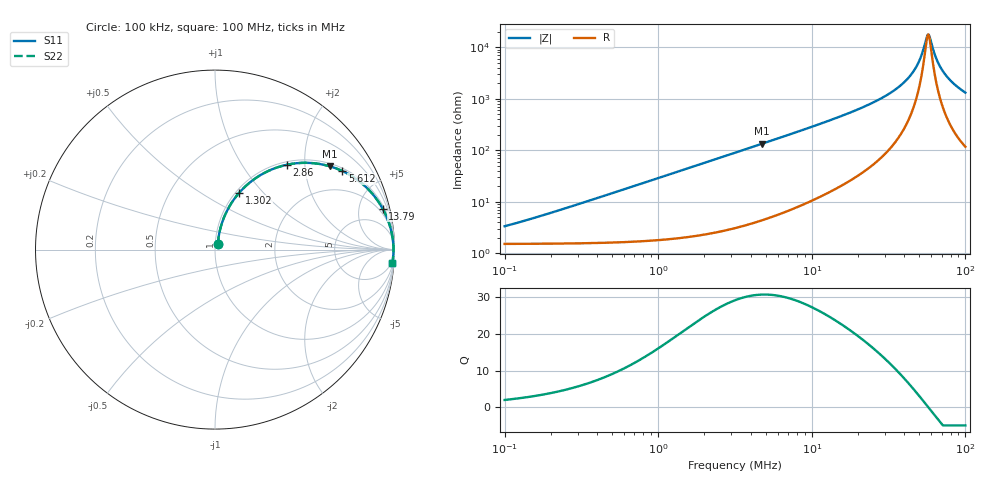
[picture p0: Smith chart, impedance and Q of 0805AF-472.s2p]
# MHz  S  MA  R  50
!Freq  MagS11  AngS11  MagS21  AngS21  MagS12  AngS12  MagS22  AngS22
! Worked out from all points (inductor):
!   801 points, 100 kHz to 100 MHz, reference 50 ohm
!   read as one part in series: L = 4.68 uH near 155.4 kHz
!   highest Q = 30.8 at 4.762 MHz (marker M1), where L = 4.49 uH
!   self-resonance near 56.89 MHz
!   S11 on the Smith chart (normalised r, x): 100 kHz: 1.03, +0.06; 1.302 MHz: 1.04, +0.75; 2.86 MHz: 1.06, +1.62; 5.612 MHz: 1.10, +3.17; 13.79 MHz: 1.33, +8.07; 100 MHz: 3, -26
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0.1  0.03284 61.4  0.9847 -1.7  0.9847 -1.7  0.03284 61.4
0.3183882  0.09249 75.3  0.9806 -5.2  0.9806 -5.2  0.09249 75.3
1.004987  0.2733 70.6  0.9451 -15.8  0.9451 -15.8  0.2733 70.6
1.302455  0.3438 67.0  0.9215 -20.1  0.9215 -20.1  0.3438 67.0
2.859717  0.619 49.8  0.7639 -38.2  0.7639 -38.2  0.619 49.8
3.172224  0.657 47.0  0.7317 -41.0  0.7317 -41.0  0.657 47.0
4.761833  0.7902 36.0  0.5877 -52.2  0.5877 -52.2  0.7902 36.0
5.611629  0.8335 31.7  0.526 -56.4  0.526 -56.4  0.8335 31.7
10.01307  0.9335 19.0  0.3261 -68.9  0.3261 -68.9  0.9335 19.0
13.78617  0.9614 13.8  0.2382 -73.9  0.2382 -73.9  0.9614 13.8
22.56254  0.9834 7.7  0.1345 -79.1  0.1345 -79.1  0.9834 7.7
31.88044  0.9904 4.5  0.07879 -80.8  0.07879 -80.8  0.9904 4.5
39.2289  0.9928 2.8  0.0497 -80.2  0.0497 -80.2  0.9928 2.8
45.43747  0.9938 1.7  0.03038 -77.4  0.03038 -77.4  0.9938 1.7
49.96911  0.9942 1.0  0.01842 -71.1  0.01842 -71.1  0.9942 1.0
55.4297  0.9944 0.2  0.007015 -37.0  0.007015 -37.0  0.9944 0.2
57.37942  0.9944 -0.0  0.005577 1.7  0.005577 1.7  0.9944 -0.0
58.88659  0.9944 -0.2  0.006571 31.8  0.006571 31.8  0.9944 -0.2
65.32168  0.9943 -1.0  0.0177 70.6  0.0177 70.6  0.9943 -1.0
71.21827  0.9939 -1.6  0.02859 76.9  0.02859 76.9  0.9939 -1.6
82.48964  0.9929 -2.7  0.04799 80.1  0.04799 80.1  0.9929 -2.7
100  0.9905 -4.3  0.0751 80.6  0.0751 80.6  0.9905 -4.3
